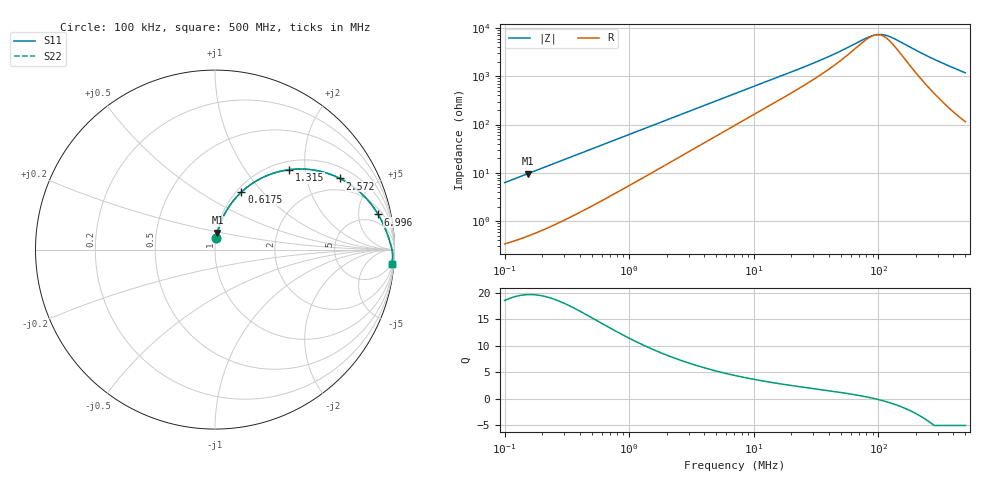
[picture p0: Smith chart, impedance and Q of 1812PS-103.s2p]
# MHz S MA R 50
!Freq  MagS11  AngS11  MagS21  AngS21  MagS12  AngS12  MagS22  AngS22
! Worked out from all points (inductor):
!   801 points, 100 kHz to 500 MHz, reference 50 ohm
!   read as one part in series: L = 9.99 uH near 104.4 kHz
!   highest Q = 19.6 at 153.1 kHz (marker M1), where L = 9.99 uH
!   self-resonance near 95.17 MHz
!   S11 on the Smith chart (normalised r, x): 100 kHz: 1.01, +0.13; 617.5 kHz: 1.05, +0.77; 1.315 MHz: 1.16, +1.64; 2.572 MHz: 1.43, +3.17; 6.996 MHz: 2.90, +8.41; 500 MHz: 3, -23
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0.1  0.06253 83.3  0.9947 -3.6  0.9947 -3.6  0.06253 83.3
0.1530906  0.09528 81.6  0.9906 -5.5  0.9906 -5.5  0.09528 81.6
0.2552035  0.1569 77.9  0.9793 -9.0  0.9793 -9.0  0.1569 77.9
0.416464  0.2491 72.1  0.9534 -14.4  0.9534 -14.4  0.2491 72.1
0.6175254  0.3527 65.3  0.9111 -20.6  0.9111 -20.6  0.3527 65.3
0.8868722  0.4693 57.4  0.8451 -27.9  0.8451 -27.9  0.4693 57.4
1.315038  0.6064 47.2  0.7375 -37.1  0.7375 -37.1  0.6064 47.2
1.716055  0.6934 40.0  0.6471 -43.6  0.6471 -43.6  0.6934 40.0
2.571771  0.8008 29.7  0.5 -52.5  0.5 -52.5  0.8008 29.7
4.108428  0.8812 19.9  0.346 -60.3  0.346 -60.3  0.8812 19.9
6.996185  0.93 12.2  0.2159 -65.1  0.2159 -65.1  0.93 12.2
7.071068  0.9307 12.0  0.2138 -65.2  0.2138 -65.2  0.9307 12.0
13.68218  0.959 6.3  0.1148 -66.0  0.1148 -66.0  0.959 6.3
29.44845  0.9746 2.7  0.05349 -60.3  0.05349 -60.3  0.9746 2.7
45.56535  0.98 1.5  0.0329 -51.9  0.0329 -51.9  0.98 1.5
87.23307  0.9857 0.2  0.0146 -11.2  0.0146 -11.2  0.9857 0.2
94.98846  0.9863 0.0  0.01374 -0.3  0.01374 -0.3  0.9863 0.0
103.4333  0.9868 -0.2  0.01347 11.6  0.01347 11.6  0.9868 -0.2
121.3434  0.9877 -0.5  0.01468 33.1  0.01468 33.1  0.9877 -0.5
137.8798  0.9884 -0.7  0.01704 46.7  0.01704 46.7  0.9884 -0.7
263.9656  0.9904 -2.3  0.04097 75.2  0.04097 75.2  0.9904 -2.3
500  0.9883 -4.8  0.08413 79.6  0.08413 79.6  0.9883 -4.8
